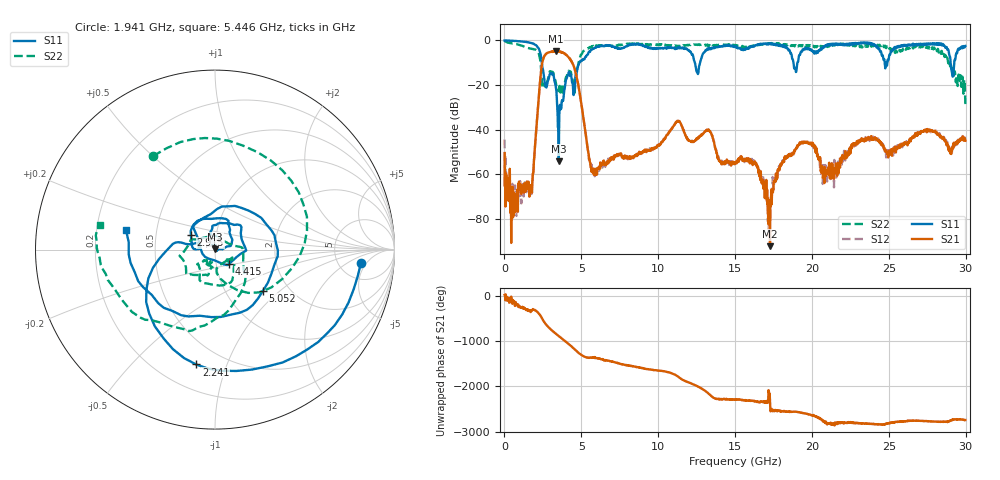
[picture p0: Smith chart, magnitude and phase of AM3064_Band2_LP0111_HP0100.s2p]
# Hz S DB R 50.0
!freq dBS11 angS11 dBS21 angS21 dBS12 angS12 dBS22 angS22
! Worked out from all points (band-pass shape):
!   1600 points, 10 MHz to 29.98 GHz, reference 50 ohm
!   highest |S21| = -4.81 dB at 3.328 GHz (marker M1); lowest = -92.2 dB at 17.27 GHz (marker M2)
!   |S21| within 3 dB of the highest: 2.545 GHz to 4.202 GHz (1.657 GHz wide, 49.1 % of centre)
!   lowest |S11| = -54.2 dB at 3.534 GHz (marker M3), VSWR 1.00, Z = 50.2 + j0.0934 ohm
!   |S11| at or under -10 dB: 2.428 GHz to 4.877 GHz (2.449 GHz wide, 67 % of centre); 12.38 GHz to 12.73 GHz (342.4 MHz wide, 2.73 % of centre); 18.8 GHz to 19.05 GHz (252.3 MHz wide, 1.33 % of centre)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
!   |S22| runs from -29.2 to -0.2 dB; largest |S21 - S12| = 0.019
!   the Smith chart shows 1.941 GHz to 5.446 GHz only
!   S11 on the Smith chart (normalised r, x): 1.941 GHz: 8.28, -3.67; 2.241 GHz: 0.36, -0.79; 2.915 GHz: 0.75, +0.13; 4.415 GHz: 1.16, -0.19; 5.052 GHz: 1.49, -0.78; 5.446 GHz: 0.33, +0.10
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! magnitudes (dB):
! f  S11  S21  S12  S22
! 10 MHz  0.0  -50.5  -44.4  -0.2
! 722.3 MHz  -0.2  -68.8  -69.2  -1.6
! 1.941 GHz  -1.8  -52.5  -52.2  -4.1
! 2.241 GHz  -3.8  -24.7  -24.6  -6.0
! 2.915 GHz  -16.0  -5.3  -5.3  -14.7
! 3.328 GHz  -20.2  -4.8  -4.9  -18.4
! 3.534 GHz  -54.2  -4.9  -5.0  -21.7
! 4.415 GHz  -19.0  -10.0  -10.0  -16.7
! 5.015 GHz  -9.3  -29.1  -28.9  -6.3
! 5.052 GHz  -9.1  -30.8  -30.7  -5.9
! 5.446 GHz  -5.9  -49.7  -50.1  -3.7
! 10 GHz  -3.6  -47.2  -46.9  -2.0
! 11.31 GHz  -3.1  -36.2  -36.2  -2.7
! 15 GHz  -2.7  -54.6  -55.1  -2.0
! 16.32 GHz  -2.2  -55.2  -54.5  -2.3
! 17.27 GHz  -1.4  -92.2  -76.8  -1.4
! 18.12 GHz  -2.8  -54.3  -54.8  -1.7
! 19.99 GHz  -4.4  -46.4  -46.8  -2.2
! 20.87 GHz  -2.3  -58.1  -55.9  -3.0
! 25 GHz  -8.3  -50.2  -49.5  -3.0
! 28.31 GHz  -1.8  -42.7  -41.7  -4.6
! 29.98 GHz  -2.5  -45.0  -44.6  -29.2
